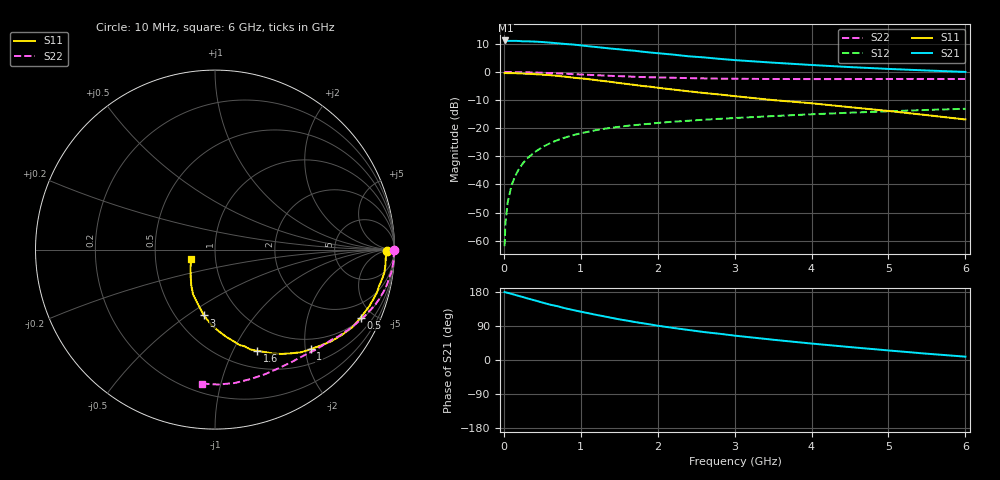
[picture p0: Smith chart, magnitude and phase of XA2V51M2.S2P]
! SIEMENS Discrete & RF Semiconductors
! BFY180
! Si NPN RF Bipolar Junction Transistor in MICRO-X
! VCE = 2.5 V  IC = 1.2 mA
! Common Emitter S-Parameters:  May  1997
# GHz  S  MA  R  50
!  f  S11  S21  S12  S22
! GHz  MAG  ANG  MAG  ANG  MAG  ANG  MAG  ANG
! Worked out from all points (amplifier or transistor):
!   36 points, 10 MHz to 6 GHz, reference 50 ohm
!   highest |S21| = 11.2 dB at 20 MHz (marker M1)
!   |S21| within 3 dB of that: start of sweep to 1.438 GHz
!   unconditionally stable (mu >= 1): 3.421 GHz to end of sweep
!   at 250 MHz: K = 0.08, MSG = 21.6 dB, |S12| = -32.4 dB
!   at 1.4 GHz: K = 0.56, MSG = 14.1 dB, |S12| = -19.8 dB
!   at 6 GHz: K = 1.07, MAG = 4.9 dB, |S12| = -13.1 dB
!   S11 on the Smith chart (normalised r, x): 10 MHz: 43, -7; 500 MHz: 1.10, -4.24; 1 GHz: 0.78, -2.11; 1.6 GHz: 0.69, -1.25; 3 GHz: 0.68, -0.58; 6 GHz: 0.76, -0.09
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0.01  0.9557 -0.4  3.552 179.5  0.0008 93.1  0.9967 -0.2
0.02  0.9592 -1.2  3.636 178.6  0.002 87.8  0.9999 -0.6
0.05  0.9526 -2.6  3.569 177.3  0.0048 85.0  0.9967 -1.4
0.1  0.9534 -5.2  3.578 174.5  0.0097 86.7  0.9964 -2.9
0.15  0.9523 -7.8  3.578 171.6  0.0144 84.6  0.9957 -4.4
0.3  0.933 -15.1  3.509 162.9  0.0287 79.8  0.9863 -8.4
0.5  0.8962 -25.0  3.41 151.7  0.0461 72.9  0.9686 -13.9
0.6  0.8785 -29.5  3.325 146.1  0.0542 70.2  0.9574 -16.4
0.7  0.8514 -34.0  3.239 141.8  0.0617 67.0  0.9449 -18.8
0.8  0.8239 -38.4  3.146 136.3  0.0687 64.3  0.9303 -21.1
1  0.7691 -46.2  2.975 127.5  0.0814 59.0  0.9034 -25.5
1.1  0.7468 -50.0  2.868 123.4  0.0867 57.0  0.8897 -27.4
1.3  0.6902 -57.4  2.688 115.3  0.0976 52.5  0.8657 -31.2
1.6  0.6113 -67.3  2.448 103.9  0.1103 48.0  0.834 -36.2
2  0.5249 -78.1  2.159 90.5  0.1243 42.5  0.801 -42.2
2.2  0.4876 -83.0  2.039 84.7  0.1307 40.0  0.7897 -45.2
2.6  0.4233 -92.2  1.818 73.8  0.1417 36.3  0.7692 -50.4
3  0.3722 -99.5  1.628 64.3  0.1519 32.7  0.7583 -55.5
3.5  0.3166 -107.8  1.465 53.5  0.1644 29.2  0.7502 -61.7
4.5  0.2368 -124.0  1.222 34.1  0.1888 21.8  0.7481 -74.7
5.5  0.1709 -143.1  1.063 16.6  0.2116 14.1  0.7521 -88.6
6  0.1431 -157.5  1.003 8.8  0.2219 10.0  0.75 -95.6
